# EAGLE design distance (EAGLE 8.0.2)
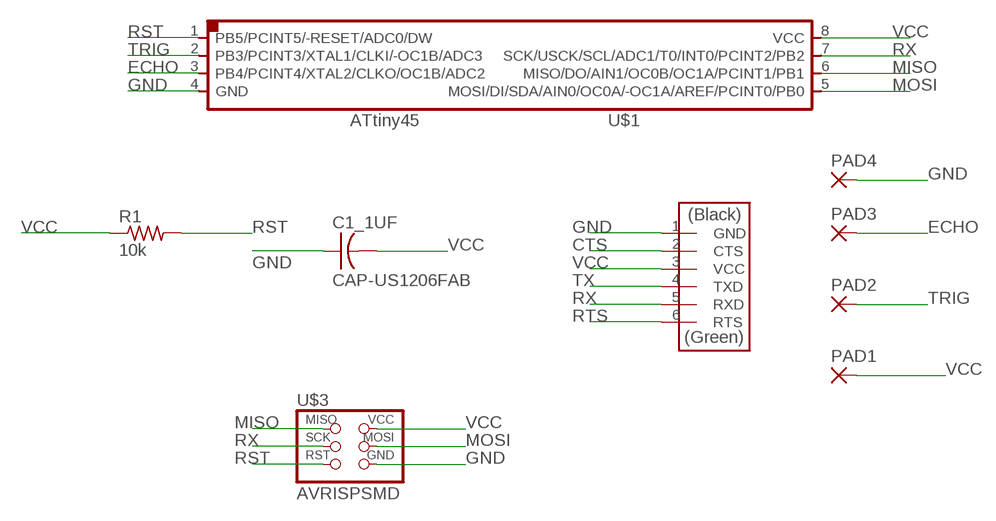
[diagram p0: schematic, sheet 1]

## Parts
C1_1UF  CAP-US1206FAB  [C1206FAB]
PAD1  SMD2  [SMD1,27-2,54]
PAD2  SMD2  [SMD1,27-2,54]
PAD3  SMD2  [SMD1,27-2,54]
PAD4  SMD2  [SMD1,27-2,54]
R1  10k  RES-US1206FAB  [R1206FAB]
U$1  ATTINY45SI  [SOIC8]
U$2  FTDI-SMD-HEADER  [1X06SMD]
U$3  AVRISPSMD  [2X03SMD]

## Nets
CTS: U$2.2(CTS)
ECHO: PAD3.1(P) U$1.3(PB4/PCINT4/XTAL2/CLKO/OC1B/ADC2)
GND: C1_1UF.1 PAD4.1(P) U$1.4(GND) U$2.1(GND) U$3.6(GND)
MISO: U$1.6(MISO/DO/AIN1/OC0B/OC1A/PCINT1/PB1) U$3.1(MISO)
MOSI: U$1.5(MOSI/DI/SDA/AIN0/OC0A/-OC1A/AREF/PCINT0/PB0) U$3.4(MOSI)
RST: R1.2 U$1.1(PB5/PCINT5/-RESET/ADC0/DW) U$3.5(RST)
RTS: U$2.6(RTS)
RX: U$1.7(SCK/USCK/SCL/ADC1/T0/INT0/PCINT2/PB2) U$2.5(RXD) U$3.3(SCK)
TRIG: PAD2.1(P) U$1.2(PB3/PCINT3/XTAL1/CLKI/-OC1B/ADC3)
TX: U$2.4(TXD)
VCC: C1_1UF.2 PAD1.1(P) R1.1 U$1.8(VCC) U$2.3(VCC) U$3.2(VCC)

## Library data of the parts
C1_1UF = fab:CAP-US
PAD1-PAD4 = wirepad:SMD2: SMD PAD
R1 = fab:RES-US: Resistor (US Symbol)
U$1 = fab:ATTINY45
U$2 = fab:FTDI-SMD-HEADER
U$3 = fab:AVRISP

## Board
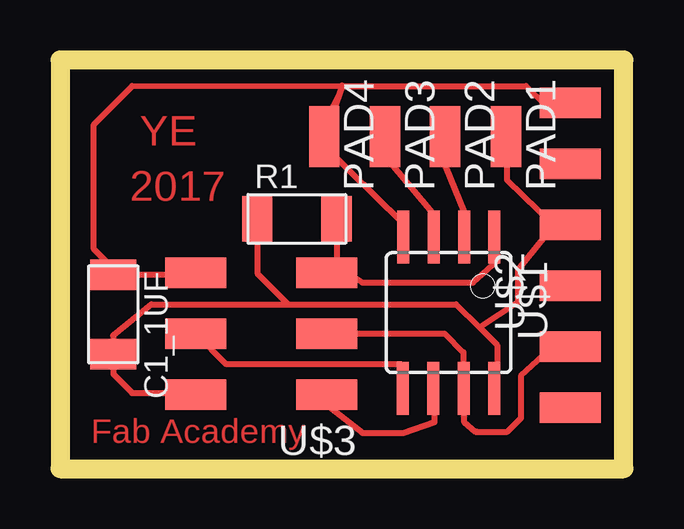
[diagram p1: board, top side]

Size 23.49 x 17.05 mm. Coordinates in mm from the lower left corner, seen from the top.
Outline: 0,0 23.49,0 23.49,17.05 0,17.05 0,0
Copper layers (1*16): Top 0.035mm / dielectric 1.5mm / Bottom 0.035mm
Design rules "default": minimum track width 10mil, minimum drill 24mil, track to track 8mil, track to pad 8mil, pad to pad 8mil, via to via 8mil, smd to smd 8mil, copper to edge 40mil, drill to drill 8mil, minimum pad ring 10mil, minimum via ring 8mil, stop-mask expansion 4mil, vias tented up to drill 0mil, thermal gap 10mil

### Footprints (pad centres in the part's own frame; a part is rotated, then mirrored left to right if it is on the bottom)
C1206FAB = smd 1.27 x 1.905: 1 -1.651,0; 2 1.651,0
SMD1,27-2,54 = smd 1.27 x 2.54: 1 0,0
R1206FAB = smd 1.27 x 1.905: 1 -1.651,0; 2 1.651,0
SOIC8 = smd 0.5 x 2.2: 1 -1.905,-3.154; 2 -0.645,-3.154; 3 0.625,-3.154; 4 1.895,-3.154; 5 1.905,3.154; 6 0.635,3.154; 7 -0.635,3.154; 8 -1.905,3.154
1X06SMD = smd 2.54 x 1.27: 1 0,6.35; 2 0,3.81; 3 0,1.27; 4 0,-1.27; 5 0,-3.81; 6 0,-6.35
2X03SMD = smd 2.54 x 1.27: 1 -2.54,2.54; 2 2.92,2.54; 3 -2.54,0; 4 2.92,0; 5 -2.54,-2.54; 6 2.92,-2.54

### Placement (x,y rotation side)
C1_1UF  2.22,6.44 270 top
PAD1  18.59,13.86 180 top
PAD2  16.05,13.86 180 top
PAD3  13.55,13.86 180 top
PAD4  11.01,13.86 180 top
R1  9.87,10.42 0 top
U$1  16.19,6.51 180 top
U$2  21.27,8.91 0 top
U$3  8.57,5.64 180 top

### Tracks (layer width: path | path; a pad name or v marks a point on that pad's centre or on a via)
ECHO
  Top 0.254: PAD3.1 13.55,13.02 15.61,10.56 15.61,9.82 U$1.3
GND
  Top 0.254: U$3.6 5.56,8.09 C1_1UF.1 2.22,8.35 1.41,9.16 1.41,14.36 3.01,15.96 11.76,15.98 PAD4.1 | PAD4.1 11.41,15.16 11.81,15.96 19.41,15.96 20.21,15.16 21.17,15.16 U$2.1 | PAD4.1 10.99,13.47 14.24,10.29 14.26,9.77 U$1.4
MISO
  Top 0.254: U$3.1 11.11,2.66 12.61,1.49 14.31,1.49 15.61,1.95 15.61,3.21 U$1.6
MOSI
  Top 0.254: U$1.5 14.29,4.29 14.21,4.36 6.93,4.36 U$3.4
RST
  Top 0.254: U$1.1 18.11,9.35 18.21,8.66 17.21,7.76 12.61,7.76 11.99,8.18 U$3.5 11.52,8.59 R1.2
RX
  Top 0.254: 16.81,3.57 U$1.7 | U$3.3 16.03,5.64 16.81,4.86 16.81,4.04 U$1.7 | U$1.7 16.82,1.96 17.31,1.55 | 17.31,1.55 17.38,1.56 | U$2.5 21.21,5.16 20.61,5.16 19.2,3.87 19.21,3.86 19.21,2.12 18.64,1.55 17.31,1.55
TRIG
  Top 0.254: PAD2.1 16.05,12.62 16.85,10.69 16.83,9.59 U$1.2
VCC
  Top 0.254: 9.51,6.86 3.81,6.86 2.21,5.56 C1_1UF.2 2.22,3.95 3.01,3.16 5.59,3.16 U$3.2 | R1.1 8.22,8.15 9.51,6.86 | 18.59,12.98 PAD1.1 18.62,12.05 20.58,10.14 | 9.51,6.86 16.51,6.86 17.48,5.9 | 17.48,5.9 18.21,5.16 18.21,3.47 U$1.8 | U$2.3 20.83,10.18 20.58,10.14 | 20.58,10.14 19.08,8.29 19.07,6.94 17.48,5.9

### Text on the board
Top: YE | 2017 | Fab Academy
